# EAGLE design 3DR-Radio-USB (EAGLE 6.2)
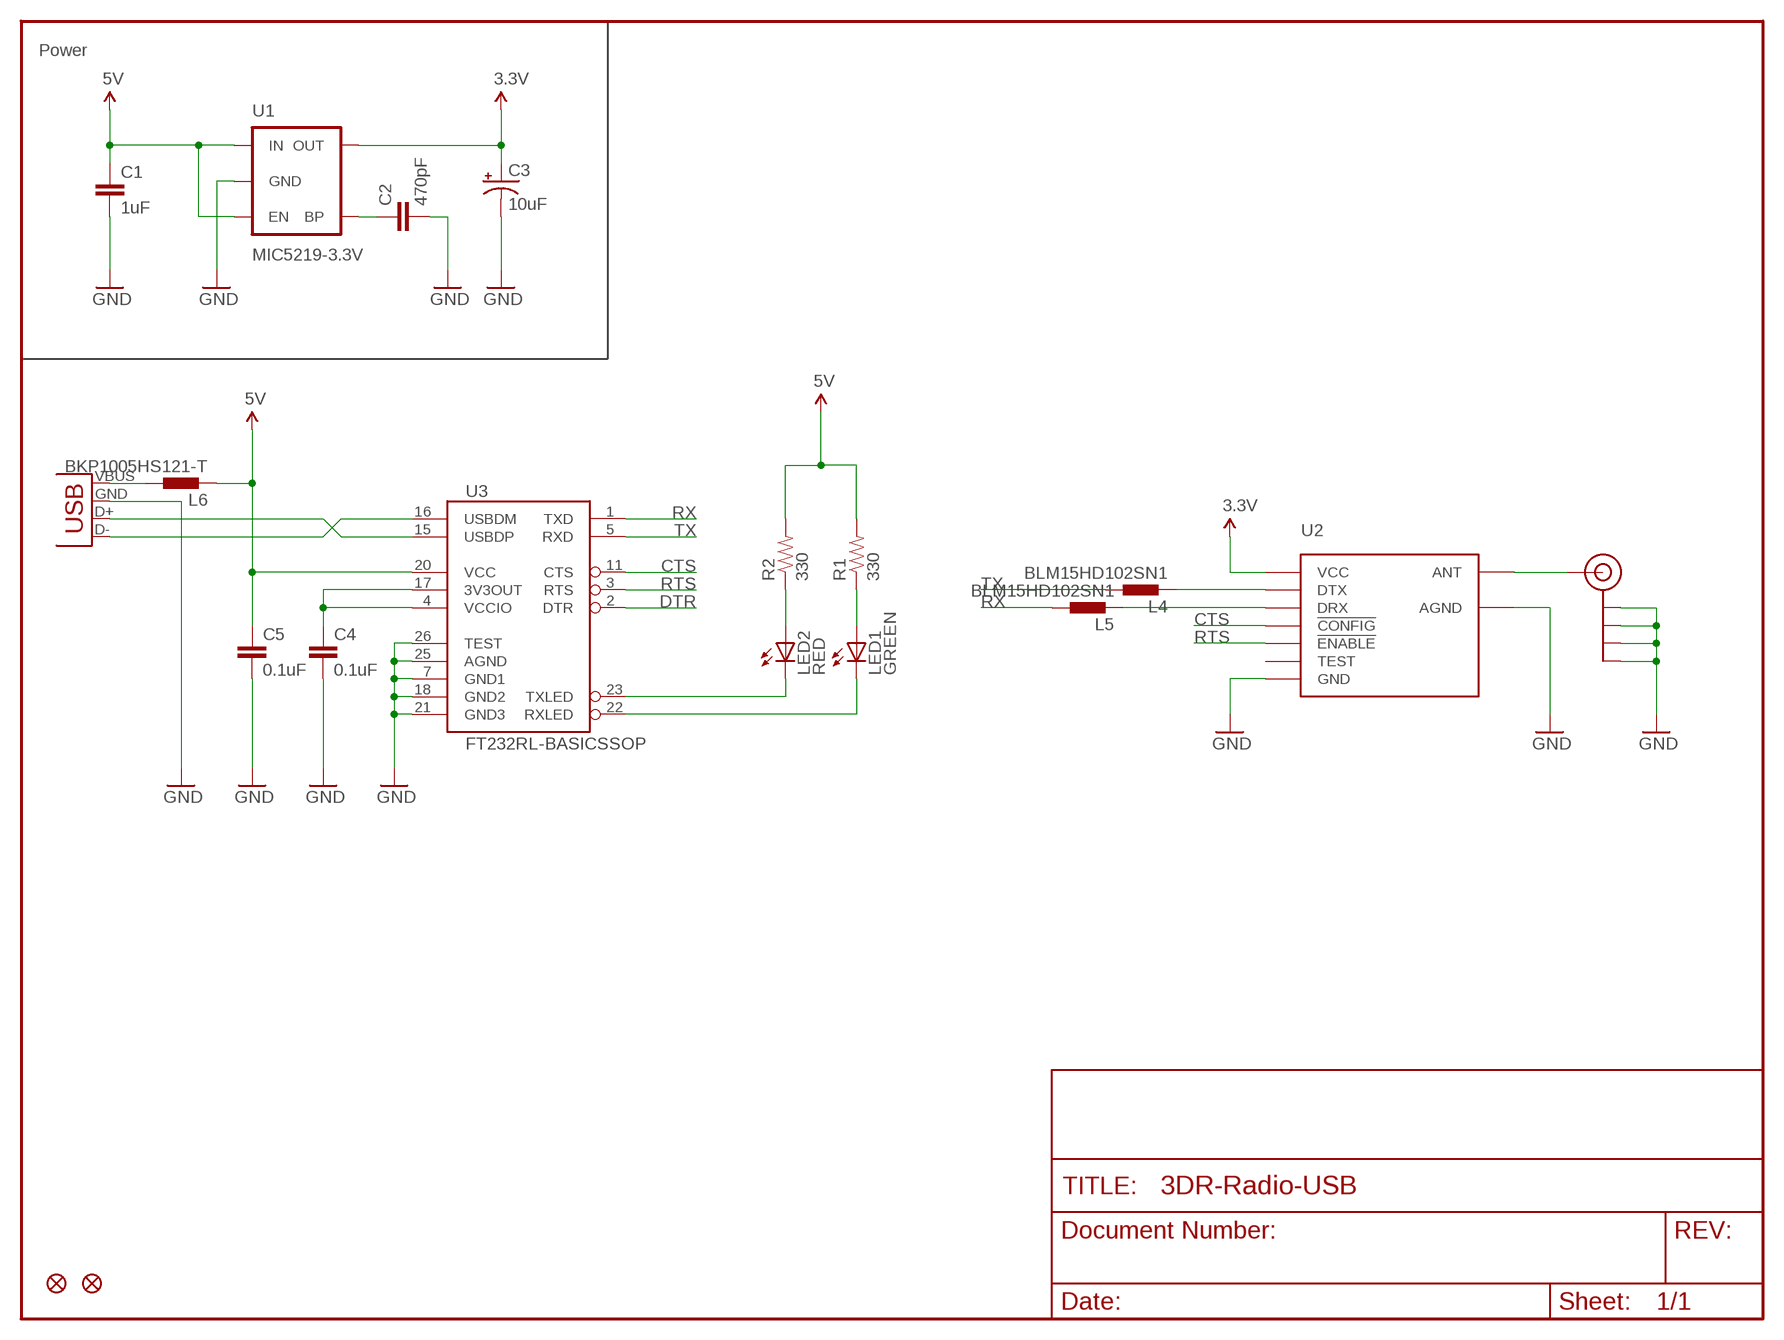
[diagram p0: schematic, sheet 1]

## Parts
C1  1uF  CAP0402-CAP  [0402-CAP]
C2  470pF  CAP0402-CAP  [0402-CAP]
C3  10uF  CAP_POL1206  [EIA3216]
C4  0.1uF  CAP0402-CAP  [0402-CAP]
C5  0.1uF  CAP0402-CAP  [0402-CAP]
J$1  SMA_EDGE  [SMA-EDGE]
JP1  FIDUCIAL1X2  [FIDUCIAL-1X2]
JP2  FIDUCIAL1X2  [FIDUCIAL-1X2]
L4  BLM15HD102SN1  INDUCTOR-0402  [0402-IND]
L5  BLM15HD102SN1  INDUCTOR-0402  [0402-IND]
L6  BKP1005HS121-T  INDUCTOR-0402  [0402-IND]
LED1  GREEN  LED0603  [LED-0603]
LED2  RED  LED0603  [LED-0603]
R1  330  RESISTOR0402-RES  [0402-RES]
R2  330  RESISTOR0402-RES  [0402-RES]
U1  MIC5219-3.3V  V_REG_LDOSMD  [SOT23-5]
U2  HM-TRPSMD  [HM-TRP-SMD]
U3  FT232RL-BASICSSOP  [SSOP28DB]
X1  USB-A-H  [USB-A-H]

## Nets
3.3V: C3.A(+) U1.5(OUT) U2.VCC
5V: C1.1 C5.1 L6.P$2 R1.2 R2.2 U1.1(IN) U1.3(EN) U3.20(VCC)
CTS: U2.!CONFIG U3.11(CTS)
DTR: U3.2(DTR)
GND: C1.2 C2.2 C3.C(-) C4.2 C5.2 J$1.GND@0(GND) J$1.GND@1(GND) J$1.GND@2(GND) J$1.GND@3(GND) U1.2(GND) U2.AGND U2.GND U3.7(GND1) U3.18(GND2) U3.21(GND3) U3.25(AGND) U3.26(TEST) X1.GND(VBUS)
N$1: J$1.SIG(SIGNAL) U2.ANT
N$2: C2.1 U1.4(BP)
N$3: C4.1 U3.4(VCCIO) U3.17(3V3OUT)
N$4: L4.P$2 U2.DTX
N$5: U3.15(USBDP) X1.D+(D-)
N$6: U3.16(USBDM) X1.D-(D+)
N$7: L5.P$2 U2.DRX
N$8: LED2.A R2.1
N$9: LED1.A R1.1
N$10: LED2.C U3.23(TXLED)
N$11: LED1.C U3.22(RXLED)
N$12: L6.P$1 X1.VBUS(GND)
RTS: U2.!ENABLE U3.3(RTS)
RX: L5.P$1 U3.1(TXD)
TX: L4.P$1 U3.5(RXD)
Unconnected: U2.TEST

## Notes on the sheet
- Power

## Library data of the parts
C1 C2 C4 C5 = SparkFun:CAP: Capacitor
C3 = SparkFun:CAP_POL: Capacitor Polarized
J$1 = 3DRobotics:SMA_EDGE: SMA Antenna Connector End launch SMA connector. The paste layer has been removed so that the connector can be hand soldered onto the board after reflow.
JP1 JP2 = SparkFun:FIDUCIAL: Fiducial Alignment Points
L4-L6 = pel_dipol_comp:INDUCTOR
LED1 LED2 = SparkFun:LED: LEDs
R1 R2 = SparkFun:RESISTOR: Resistor
U1 = SparkFun:V_REG_LDO: Voltage Regulator LDO Standard 150mA LDO voltage regulator in SOT-23 layout. Micrel part MIC5205. BP (by-pass) pin is used to lower output noise with 470pF cap.
U2 = 3DRobotics:HM-TRP: HM-TRP Series 100mW Transceiver module HM-TRP series is a low cost, high performance transparent FSK transceiver with operating at 433/470/868/915 MHz. It features small size, high output power, high sensitivity, long transmission distance and high communication data rate with auto set up for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
U3 = SparkFun:FT232RL-BASIC: USB UART This is the simplified version of the FT232RL unit. Only what you need, nothing you don't. Spark Fun Electronics SKU : COM-00650
X1 = SparkFun:USB: USB Connectors USB-B-PTH is fully proven SKU : PRT-00139 USB-miniB is fully proven SKU : PRT-00587 USB-A-PCB is untested. USB-A-H is throughly reviewed, but untested. Spark Fun Electronics SKU : PRT-00437 USB-B-SMT is throughly reviewed, but untested. Needs silkscreen touching up. USB-A-S has not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

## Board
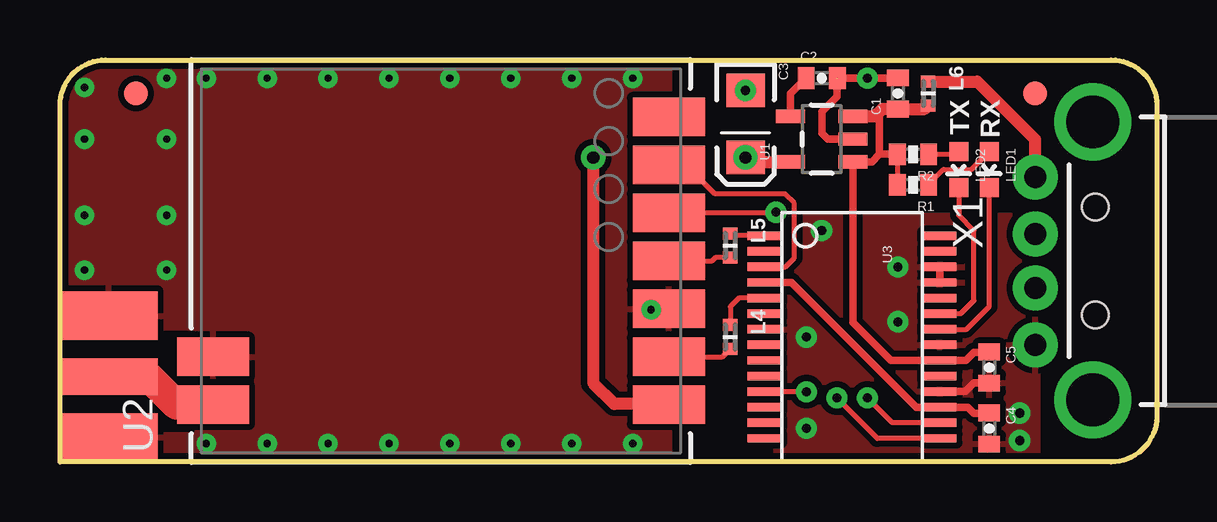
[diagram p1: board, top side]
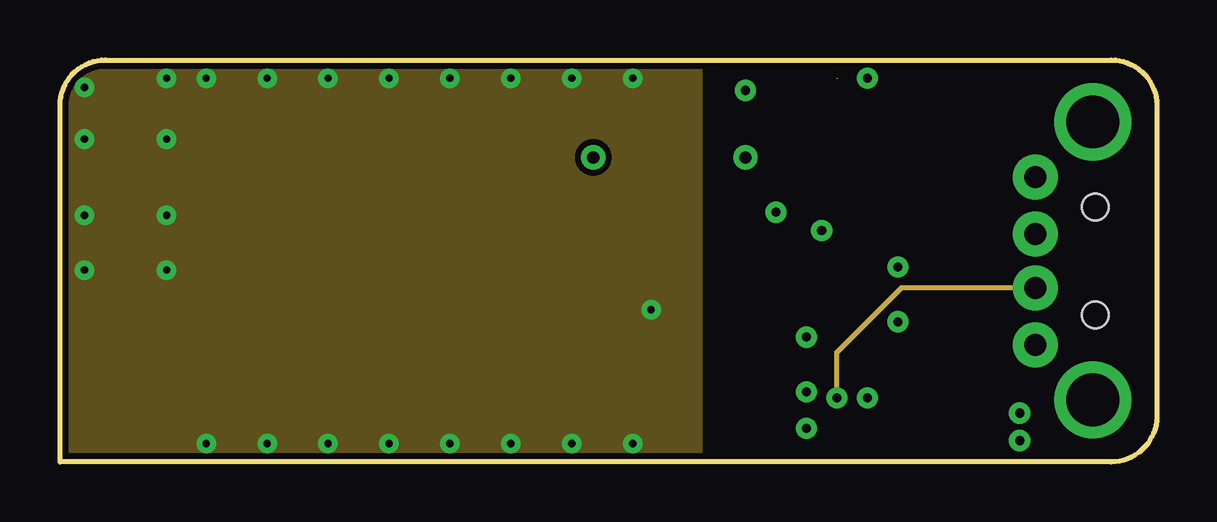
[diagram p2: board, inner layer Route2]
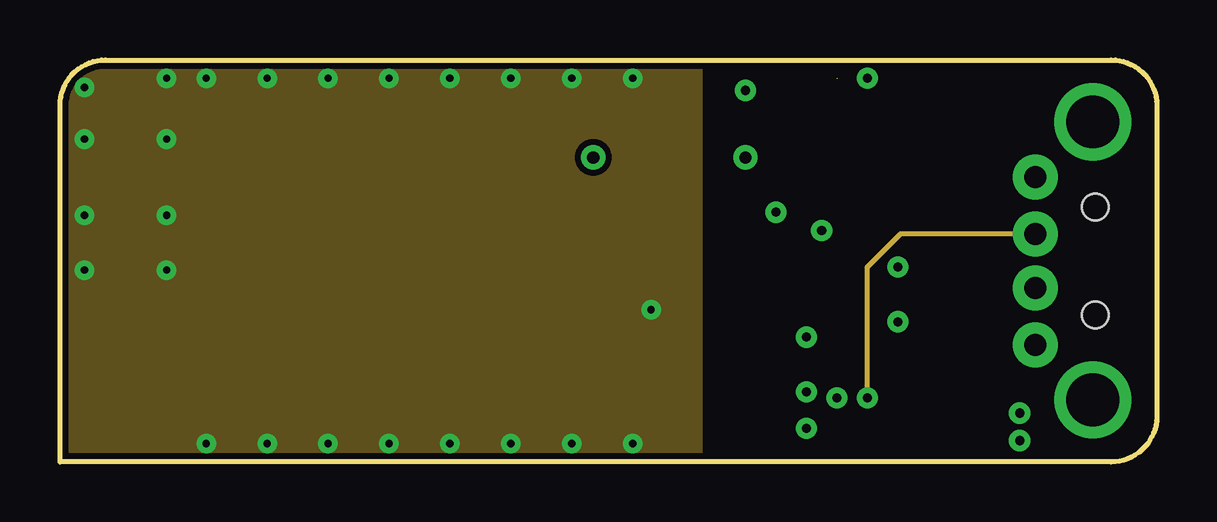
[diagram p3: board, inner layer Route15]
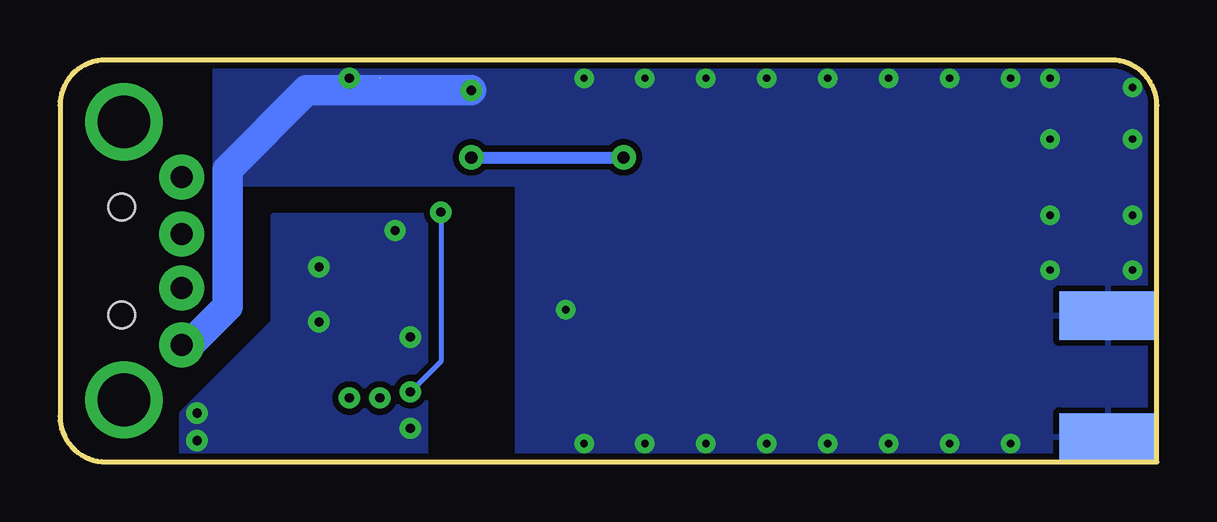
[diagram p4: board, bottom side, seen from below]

Size 45.72 x 16.76 mm. Coordinates in mm from the lower left corner, seen from the top.
Outline: 0,0 0,14.86 arc-90 1.91,16.76 43.81,16.76 arc-90 45.72,14.86 45.72,1.9 arc-90 43.81,0 0,0
Copper layers (1*2*15*16): Top 0.035mm / dielectric 0.5mm / Route2 0.035mm / dielectric 0.5mm / Route15 0.035mm / dielectric 0.5mm / Bottom 0.035mm
Design rules: minimum track width 7mil, minimum drill 10mil, track to track 7mil, track to pad 7mil, pad to pad 7mil, via to via 7mil, smd to smd 0mil, copper to edge 10mil, drill to drill 8mil, minimum pad ring 12mil, minimum via ring 10mil, stop-mask expansion 4mil, vias tented up to drill 25mil, thermal gap 10mil

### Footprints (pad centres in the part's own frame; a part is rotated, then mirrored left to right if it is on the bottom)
0402-CAP = smd 0.7 x 0.9: 1 -0.65,0; 2 0.65,0
EIA3216 = smd 1.4 x 1.6: A 1.4,0; C -1.4,0
SMA-EDGE = smd 2.032 x 4.064: GND@0 -2.54,0; GND@1 2.54,0 | smd 2.032 x 4.064 bottom: GND@2 -2.54,0; GND@3 2.54,0 | smd 1.524 x 4.064: SIG 0,0
FIDUCIAL-1X2 = smd 1 x 1: 1 0,0
0402-IND = smd 0.5 x 0.6: P$1 -0.5,0; P$2 0.5,0
LED-0603 = smd 0.8 x 0.8: A 0,-0.75; C 0,0.75
0402-RES = smd 0.7 x 0.9: 1 -0.65,0; 2 0.65,0
SOT23-5 = smd 0.55 x 1.2: 1 -0.95,-1.3; 2 0,-1.3; 3 0.95,-1.3; 4 0.95,1.3; 5 -0.95,1.3
HM-TRP-SMD = smd 1.6 x 3: !CONFIG 2,-9.5; !ENABLE 4,-9.5; AGND -4,9.5; ANT -6,9.5; DRX 0,-9.5; DTX -4,-9.5; GND -2,-9.5; TEST 6,-9.5; VCC -6,-9.5
SSOP28DB = smd 0.348 x 1.397: 1 -4.225,-3.656; 2 -3.575,-3.656; 3 -2.925,-3.656; 4 -2.275,-3.656; 5 -1.625,-3.656; 6 -0.975,-3.656; 7 -0.325,-3.656; 8 0.325,-3.656; 9 0.975,-3.656; 10 1.625,-3.656; 11 2.275,-3.656; 12 2.925,-3.656; 13 3.575,-3.656; 14 4.225,-3.656; 15 4.225,3.656; 16 3.575,3.656; 17 2.925,3.656; 18 2.275,3.656; 19 1.625,3.656; 20 0.975,3.656; 21 0.325,3.656; 22 -0.325,3.656; 23 -0.975,3.656; 24 -1.625,3.656; 25 -2.275,3.656; 26 -2.925,3.656; 27 -3.575,3.656; 28 -4.225,3.656
USB-A-H = drill 0.914 pad 1.88: D+ 2.4,1.127; D- 2.4,-1.127; GND 2.4,3.5; VBUS 2.4,-3.5 | drill 2.2: GND2 0,-5.8; GND3 0,5.8 | hole 1.1: -0.1,2.25; -0.1,-2.25

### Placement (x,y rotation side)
C1  34.92,15.37 90 top
C2  31.75,16 0 top
C3  28.57,14.1 270 top
C4  38.73,1.4 270 top
C5  38.73,3.94 270 top
J$1  2.03,3.56 90 top
JP1  40.64,15.37 0 top
JP2  3.17,15.37 0 top
L4  27.94,5.21 270 top
L5  27.94,9.02 270 top
L6  36.2,15.37 270 top
LED1  38.73,12.19 180 top
LED2  37.47,12.19 180 top
R1  35.56,11.56 180 top
R2  35.56,12.83 180 top
U1  31.75,13.46 90 top
U2  15.88,8.38 90 top
U3  33.02,5.21 270 top
X1  43.05,8.38 180 top

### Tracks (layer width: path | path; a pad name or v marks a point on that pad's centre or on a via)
3.3V  (via drill 0.51)
  Top 0.508: U2.VCC 25.41,2.41 23.11,2.41 22.23,3.3 v22.23,12.7 | U1.5 29.39,12.51 C3.A
  Bottom 0.508: C3.A v22.23,12.7
  other vias: 28.57,12.7
5V
  Top 0.203: R2.2 R1.2
  Top 0.305: C5.1 38.72,4.57 38.1,4.57 37.76,4.23 U3.20 34.63,4.23 33.05,5.81 U1.1 33.85,12.51 34.16,12.83 | 34.16,12.83 34.16,14.73 34.91,14.73 C1.1 | R2.2 34.16,12.83
  Top 0.508: U1.3 33.97,14.41 34.27,14.72 C1.1 36.05,14.72 L6.P$2
CTS  (via drill 0.38)
  Top 0.203: U2.!CONFIG 29.81,10.38 v29.84,10.41 | U3.11 v31.1,2.93 v31.11,2.92
  Bottom 0.203: v29.84,10.41 29.84,4.19 v31.11,2.92
GND  (via drill 0.3, 0.38)  (1 unrouted)
  Top 0.305: U3.18 37.73,2.93 38.1,3.3 C5.2 | U3.25 U3.26 | U1.2 32,13.46 31.75,13.72 31.75,14.61 32.38,15.24 32.38,16 v33.66,16 C1.2 | C3.C
  Bottom 0.305: v33.66,16 34.04,16 34.29,15.75
  Bottom 1.27: C3.C 35.43,15.49 38.73,12.19 38.73,6.48 40.33,4.88 X1.GND
  other vias: 1.02,15.62 4.45,16 6.1,16 8.64,16 11.18,16 13.72,16 16.26,16 18.8,16 21.34,16 1.02,10.29 1.02,13.46 1.02,8 4.45,8 4.45,10.29 4.45,13.46 6.1,0.76 8.64,0.76 11.18,0.76 13.72,0.76 16.26,0.76 18.8,0.76 21.34,0.76 24.64,6.35 23.88,16 23.88,0.76 34.92,8.13 31.11,5.21 34.92,5.84 31.75,9.65 31.11,1.4 40.01,2.03 40.01,0.89 28.57,15.49
  pour Top (isolate 0.254): 5.71,-1.14 5.71,19.18 25.4,19.18 25.4,-1.14
  pour Bottom (isolate 0.254): 5.71,-1.14 5.71,20.45 26.67,20.45 26.67,-1.14
  pour Top (isolate 0.254): 5.71,-1.14 -0.64,-1.14 -0.64,1.14 5.71,1.14
  pour Top (isolate 0.254): -0.64,5.59 5.71,5.59 5.71,17.91 -0.64,17.91
  pour Bottom (isolate 0.254): 5.71,17.91 -1.27,17.91 -1.27,4.83 5.84,4.83
  pour Bottom (isolate 0.254): -1.27,-1.14 -1.27,5.46 5.71,5.46 5.71,-1.14
  pour Route2 (isolate 0.254): 0,-0.51 0,21.08 26.67,20.45 26.67,-1.14
  pour Route15 (isolate 0.254): 0,-0.51 0,22.35 26.67,22.35 26.67,-0.51
  pour Top (isolate 0.254): 29.84,-1.78 29.84,10.29 40.77,10.29 40.77,-1.78
  pour Bottom (isolate 0.254): 40.64,-2.41 40.64,2.03 36.83,5.84 36.83,10.29 30.48,10.29 30.48,-2.41
  pour Bottom (isolate 0.254): 26.67,19.18 26.67,11.56 39.24,11.56 39.24,19.18
N$1
  Top 1.219: J$1.SIG 3.68,3.56 4.86,2.38 U2.ANT
N$2
  Top 0.305: U1.4 30.45,15.35 C2.1
N$3
  Top 0.305: U3.4 30.49,7.48 35.69,2.28 U3.17 37.85,2.28 38.1,2.03 38.72,2.03 C4.1
N$4
  Top 0.203: U2.DTX 27.61,4.38 L4.P$2
N$5  (via drill 0.38)
  Top 0.203: U3.15 34.07,0.98 v32.38,2.67
  Route2 0.203: v32.38,2.67 32.38,4.57 35.07,7.25 X1.D+
N$6  (via drill 0.38)
  Top 0.203: U3.16 34.69,1.63 v33.66,2.67
  Route15 0.203: v33.66,2.67 33.66,8.13 35.04,9.51 X1.D-
N$7
  Top 0.203: U2.DRX 27.18,8.38 27.31,8.52 L5.P$2
N$8
  Top 0.203: R2.1 37.35,12.83 LED2.A
N$9
  Top 0.203: R1.1 36.21,11.57 36.83,12.19 37.98,12.19 LED1.A
N$10
  Top 0.203: U3.23 37.55,6.18 38.1,6.73 38.1,9.65 37.47,10.29 LED2.C
N$11
  Top 0.203: U3.22 37.79,5.53 38.73,6.48 LED1.C
N$12
  Top 0.508: X1.VBUS 40.65,13.45 38.23,15.87 L6.P$1
RTS
  Top 0.203: U2.!ENABLE 26.1,12.38 27.3,11.18 30.23,11.18 30.61,10.8 30.61,8.51 30.23,8.13 U3.3
RX
  Top 0.203: U3.1 28.02,9.43 L5.P$1
TX
  Top 0.203: U3.5 28.3,6.83 27.94,6.48 L4.P$1

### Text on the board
tPlace: TX | RX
